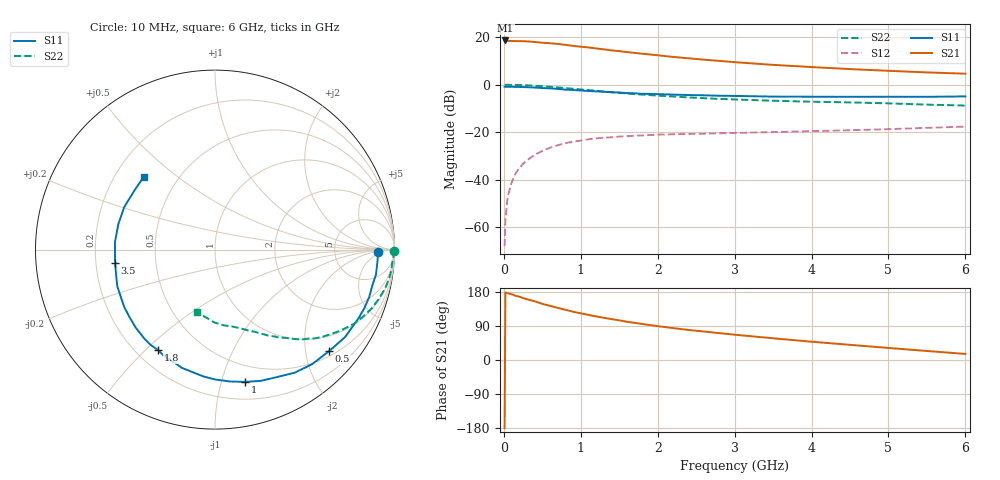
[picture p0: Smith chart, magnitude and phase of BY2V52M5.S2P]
! SIEMENS Small Signal Semiconductors
! BFY420
! Si NPN RF SIEGET Grounded Emitter Transistor in MICRO-X
! VCE = 2.5 V  IC = 2.5 mA
! Common Emitter S-Parameters:  October  1996
# GHz  S  MA  R  50
!  f  S11  S21  S12  S22
! GHz  MAG  ANG  MAG  ANG  MAG  ANG  MAG  ANG
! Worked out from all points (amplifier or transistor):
!   36 points, 10 MHz to 6 GHz, reference 50 ohm
!   highest |S21| = 18.6 dB at 20 MHz (marker M1)
!   |S21| within 3 dB of that: start of sweep to 1.114 GHz
!   unconditionally stable (mu >= 1): 3.812 GHz to end of sweep
!   at 250 MHz: K = 0.06, MSG = 25.8 dB, |S12| = -33.3 dB
!   at 1.4 GHz: K = 0.34, MSG = 18.3 dB, |S12| = -22.1 dB
!   at 6 GHz: K = 1.22, MAG = 8.3 dB, |S12| = -17.6 dB
!   S11 on the Smith chart (normalised r, x): 10 MHz: 20, -4; 500 MHz: 0.61, -2.50; 1 GHz: 0.35, -1.19; 1.8 GHz: 0.29, -0.55; 3.5 GHz: 0.28, -0.06; 6 GHz: 0.32, +0.38
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0.01  0.9064 -1.0  8.517 -179.8  0.0004 80.2  0.9968 -0.4
0.02  0.9079 -1.8  8.541 178.3  0.0014 84.9  0.9938 -0.8
0.05  0.9076 -4.4  8.343 176.1  0.0044 85.3  0.995 -2.1
0.1  0.9075 -8.8  8.338 173.8  0.0086 87.1  0.99 -4.3
0.15  0.8989 -13.0  8.288 169.5  0.0134 81.9  0.9892 -6.6
0.2  0.8989 -17.1  8.25 167.1  0.0176 80.6  0.9853 -8.6
0.3  0.8864 -25.6  8.164 160.3  0.0256 75.8  0.9724 -12.9
0.4  0.8733 -33.9  7.933 155.0  0.0334 71.7  0.9522 -16.9
0.5  0.8511 -41.6  7.65 148.1  0.0405 66.7  0.9311 -20.8
0.7  0.8173 -57.0  7.219 137.6  0.0533 58.9  0.8791 -27.9
0.9  0.7744 -70.8  6.571 127.4  0.0635 51.5  0.8222 -33.8
1  0.7555 -77.3  6.312 123.2  0.0668 48.7  0.7953 -36.5
1.1  0.739 -83.7  6.088 119.1  0.0709 46.0  0.7695 -39.2
1.4  0.6938 -100.5  5.274 107.8  0.0783 39.2  0.6987 -45.7
1.6  0.6662 -110.7  4.862 100.9  0.0827 35.6  0.6546 -49.3
1.8  0.6437 -119.5  4.484 95.0  0.0857 32.7  0.6204 -52.3
2.2  0.62 -135.4  3.844 84.2  0.0904 27.9  0.5651 -58.1
2.8  0.5862 -154.1  3.175 70.9  0.0951 23.7  0.5025 -65.1
3.5  0.5621 -172.3  2.617 57.3  0.1007 21.2  0.4603 -72.2
4.5  0.557 165.2  2.133 40.0  0.1101 18.7  0.4246 -83.4
5.5  0.5565 144.0  1.815 23.8  0.1237 16.6  0.3813 -97.5
6  0.5676 134.5  1.707 16.0  0.1313 14.9  0.3639 -105.8
